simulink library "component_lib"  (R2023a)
settings: Solver=VariableStepAuto  StartTime=0.0  StopTime=10.0  RelTol=1e-3
undefined symbols (not defined in the file or in its folder): component_lib, ECCV_r, KoblenzTrier, mm, par, param_TD04, R1234yf_ph, SigIdentifier, Systems, TH0023_WP120, Thermal, V_nom
libraries: base_lib x166, $bdroot x164, simulink x2, slpidlib x1
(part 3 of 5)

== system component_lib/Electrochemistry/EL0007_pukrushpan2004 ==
  I [A] : Inport
  p_an [Pa x 4] : Inport  Port=2
  p_ca [Pa x 4] : Inport  Port=3
  T_an [K] : Inport  Port=4
  T_ca [K] : Inport  Port=5
  T_fc [K] : Inport  Port=6
  Demux : Demux
  Demux1 : Demux
  F0003_diffusiveFlow.m : base_lib/F0003_pukrushpan2004/F0003_diffusiveFlow.m  SystemSampleTime=-1  VariantActivationTime=update diagram  Latency=0  AutoFrameSizeCalculation=off
  F0003_dragFlow.m : base_lib/F0003_pukrushpan2004/F0003_dragFlow.m  SystemSampleTime=-1  VariantActivationTime=update diagram  Latency=0  AutoFrameSizeCalculation=off
  F0003_outputVoltage.m : base_lib/F0003_pukrushpan2004/F0003_outputVoltage.m  SystemSampleTime=-1  VariantActivationTime=update diagram  Latency=0  AutoFrameSizeCalculation=off
  F0003_reactionFlow.m : base_lib/F0003_pukrushpan2004/F0003_reactionFlow.m  SystemSampleTime=-1  VariantActivationTime=update diagram  Latency=0  AutoFrameSizeCalculation=off
  F0003_vaporActivity.m : base_lib/F0003_pukrushpan2004/F0003_vaporActivity.m  SystemSampleTime=-1  VariantActivationTime=update diagram  Latency=0  AutoFrameSizeCalculation=off
  F0003_vaporActivity.m1 : base_lib/F0003_pukrushpan2004/F0003_vaporActivity.m  SystemSampleTime=-1  VariantActivationTime=update diagram  Latency=0  AutoFrameSizeCalculation=off
  F0003_waterContent.m : base_lib/F0003_pukrushpan2004/F0003_waterContent.m  SystemSampleTime=-1  VariantActivationTime=update diagram  Latency=0  AutoFrameSizeCalculation=off
  F0003_waterContent.m1 : base_lib/F0003_pukrushpan2004/F0003_waterContent.m  SystemSampleTime=-1  VariantActivationTime=update diagram  Latency=0  AutoFrameSizeCalculation=off
  F0010_vaporSaturationPressure.m : base_lib/F0010_gasFlow/F0010_vaporSaturationPressure.m  SystemSampleTime=-1  VariantActivationTime=update diagram  Latency=0  AutoFrameSizeCalculation=off
  F0010_vaporSaturationPressure.m1 : base_lib/F0010_gasFlow/F0010_vaporSaturationPressure.m  SystemSampleTime=-1  VariantActivationTime=update diagram  Latency=0  AutoFrameSizeCalculation=off
  F0010_vaporSaturationPressure.m2 : base_lib/F0010_gasFlow/F0010_vaporSaturationPressure.m  SystemSampleTime=-1  VariantActivationTime=update diagram  Latency=0  AutoFrameSizeCalculation=off
  Gain : Gain  Gain=1/2
  Mux : Mux
  Saturation : Saturate  UpperLimit=inf  LowerLimit=0.01
  Saturation1 : Saturate  UpperLimit=inf  LowerLimit=100
  Saturation2 : Saturate  UpperLimit=inf  LowerLimit=100
  Sum : Sum  Inputs=+|+
  Sum1 : Sum  Inputs=|+-
  Sum2 : Sum  Inputs=|++
  Sum4 : Sum  Inputs=|++
  V [V] : Outport
  W_an [kg/s] : Outport  Port=2
  W_ca [kg/s] : Outport  Port=3
  lam [-] : Outport  Port=4
  Q_gen [J/s] : Outport  Port=5
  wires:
  I [A]/1 -> [I], F0003_reactionFlow.m/1, F0003_outputVoltage.m/1
  F0003_outputVoltage.m/1 -> Saturation/1
  F0003_outputVoltage.m/2 -> Q_gen [J/s]/1
  T_fc [K]/1 -> F0003_diffusiveFlow.m/4, F0010_vaporSaturationPressure.m2/1, F0003_outputVoltage.m/6
  F0010_vaporSaturationPressure.m2/1 -> F0003_outputVoltage.m/4
  F0010_vaporSaturationPressure.m1/1 -> F0003_vaporActivity.m/2
  F0010_vaporSaturationPressure.m/1 -> F0003_vaporActivity.m1/2
  T_an [K]/1 -> F0010_vaporSaturationPressure.m1/1
  T_ca [K]/1 -> F0010_vaporSaturationPressure.m/1
  Demux/3 -> F0003_vaporActivity.m/1
  Demux1/3 -> F0003_vaporActivity.m1/1
  p_an [Pa x 4]/1 -> Demux/1, Saturation1/1
  p_ca [Pa x 4]/1 -> Demux1/1, Saturation2/1
  F0003_vaporActivity.m/1 -> F0003_waterContent.m/1
  F0003_vaporActivity.m1/1 -> F0003_waterContent.m1/1
  F0003_waterContent.m/1 -> Sum/1, F0003_diffusiveFlow.m/1
  F0003_waterContent.m1/1 -> F0003_diffusiveFlow.m/3, Sum/2
  F0003_reactionFlow.m/1 -> Sum1/1
  Sum1/1 -> W_an [kg/s]/1
  F0003_reactionFlow.m/2 -> Sum2/1
  Sum2/1 -> W_ca [kg/s]/1
  [I] -> F0003_dragFlow.m/1
  F0003_diffusiveFlow.m/1 -> Sum4/1
  F0003_dragFlow.m/1 -> Sum4/2
  Mux/1 -> Sum1/2, Sum2/2
  Sum/1 -> Gain/1
  Sum4/1 -> Mux/3
  Saturation/1 -> V [V]/1
  Saturation1/1 -> F0003_outputVoltage.m/2
  Saturation2/1 -> F0003_outputVoltage.m/3
  Gain/1 -> lam [-]/1, F0003_outputVoltage.m/5, F0003_dragFlow.m/2, F0003_diffusiveFlow.m/2

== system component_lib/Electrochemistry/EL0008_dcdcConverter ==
  I_in [A] : Inport
  V_in [V] : Inport  Port=2
  V_bus [V] : Inport  Port=3
  F0020_dcdcConverter.m : base_lib/F0020_dcdcConverter/F0020_dcdcConverter.m  SystemSampleTime=-1  VariantActivationTime=update diagram  Latency=0  AutoFrameSizeCalculation=off
  Terminator : Terminator
  Terminator1 : Terminator
  I_bus [A] : Outport
  Q_gen [J/s] : Outport  Port=2
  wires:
  V_bus [V]/1 -> F0020_dcdcConverter.m/1
  V_in [V]/1 -> F0020_dcdcConverter.m/2
  I_in [A]/1 -> F0020_dcdcConverter.m/3
  F0020_dcdcConverter.m/2 -> I_bus [A]/1
  F0020_dcdcConverter.m/1 -> Terminator/1
  F0020_dcdcConverter.m/4 -> Q_gen [J/s]/1
  F0020_dcdcConverter.m/3 -> Terminator1/1

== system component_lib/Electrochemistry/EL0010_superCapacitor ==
  dI [A] : Inport
  Gain : Gain  Gain=1/C
  Integrator Limited : Integrator  InitialCondition=V_bus0  LimitOutput=on  LowerSaturationLimit=0
  V_bus [V] : Outport
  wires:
  Integrator Limited/1 -> V_bus [V]/1
  dI [A]/1 -> Gain/1
  Gain/1 -> Integrator Limited/1

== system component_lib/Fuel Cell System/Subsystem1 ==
  note: Rolling Fuel Consumption Calculation [kg/100km]
  In1 : Inport
  Add1 : Sum
  Constant6 : Constant
  Constant7 : Constant  Value=100e3
  Demux : Demux
  Divide : Product  Inputs=**/
  Gain1 : Gain  Gain=-1
  Integrator : Integrator
  SC0002_signalRead11 : $bdroot/Data & Control/SC0002_signalRead  SigName=fuelConsumption
  SC0002_signalRead5 : $bdroot/Data & Control/SC0002_signalRead  SigName=hydrogenFlow
  SC0003_signalWrite1 : $bdroot/Data & Control/SC0003_signalWrite  SigName=distance
  Terminator : Terminator
  Terminator1 : Terminator
  Terminator2 : Terminator
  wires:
  Integrator/1 -> Divide/1
  Constant7/1 -> Divide/2
  SC0003_signalWrite1/1 -> Add1/1
  Demux/1 -> Gain1/1
  Add1/1 -> Divide/3
  Constant6/1 -> Add1/2
  Divide/1 -> SC0002_signalRead11/1
  Gain1/1 -> SC0002_signalRead5/1, Integrator/1
  In1/1 -> Demux/1
  Demux/3 -> Terminator1/1
  Demux/4 -> Terminator2/1
  Demux/2 -> Terminator/1

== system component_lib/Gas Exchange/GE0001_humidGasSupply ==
  Constant : Constant  Value=par.p_tot
  Constant1 : Constant  Value=par.RH
  Constant2 : Constant  Value=par.T
  Constant3 : Constant  Value=par.x_H2
  Constant4 : Constant  Value=par.x_O2
  F0010_pressureSupply.m : base_lib/F0010_gasFlow/F0010_pressureSupply.m  SystemSampleTime=-1  VariantActivationTime=update diagram  Latency=0  AutoFrameSizeCalculation=off
  F0010_vaporSaturationPressure.m : base_lib/F0010_gasFlow/F0010_vaporSaturationPressure.m  SystemSampleTime=-1  VariantActivationTime=update diagram  Latency=0  AutoFrameSizeCalculation=off
  p (p x 4) : Outport
  T [K] : Outport  Port=2
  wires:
  Constant2/1 -> T [K]/1, F0010_vaporSaturationPressure.m/1
  Constant/1 -> F0010_pressureSupply.m/1
  F0010_vaporSaturationPressure.m/1 -> F0010_pressureSupply.m/5
  Constant1/1 -> F0010_pressureSupply.m/4
  Constant3/1 -> F0010_pressureSupply.m/2
  Constant4/1 -> F0010_pressureSupply.m/3
  F0010_pressureSupply.m/1 -> p (p x 4)/1

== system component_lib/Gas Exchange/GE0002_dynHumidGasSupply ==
  T [K] : Inport
  p_ref [Pa] : Inport  Port=2
  RH [-] : Inport  Port=3
  Constant : Constant  Value=x_H2_dry
  Constant1 : Constant  Value=x_O2_dry
  F0010_pressureSupply.m : base_lib/F0010_gasFlow/F0010_pressureSupply.m  SystemSampleTime=-1  VariantActivationTime=update diagram  Latency=0  AutoFrameSizeCalculation=off
  F0010_vaporSaturationPressure.m : base_lib/F0010_gasFlow/F0010_vaporSaturationPressure.m  SystemSampleTime=-1  VariantActivationTime=update diagram  Latency=0  AutoFrameSizeCalculation=off
  p (p x 4) : Outport
  T_out [K] : Outport  Port=2
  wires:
  p_ref [Pa]/1 -> F0010_pressureSupply.m/1
  T [K]/1 -> F0010_vaporSaturationPressure.m/1, T_out [K]/1
  F0010_vaporSaturationPressure.m/1 -> F0010_pressureSupply.m/5
  RH [-]/1 -> F0010_pressureSupply.m/4
  F0010_pressureSupply.m/1 -> p (p x 4)/1
  Constant/1 -> F0010_pressureSupply.m/2
  Constant1/1 -> F0010_pressureSupply.m/3

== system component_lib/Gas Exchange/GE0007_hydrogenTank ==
  W_H2 [kg/s] : Inport
  Actuator dynamics : TransferFcn  Denominator=[0.1 1]
  Constant : Constant  Value=0
  Constant2 : Constant  Value=par.V
  Constant3 : Constant  Value=par.T_tank
  Constant4 : Constant  Value=0
  Constant5 : Constant  Value=par.m0
  Constant6 : Constant  Value=par.m0
  Constant7 : Constant  Value=par.M_j(1)
  Constant8 : Constant  Value=par.init_SOC
  Constant9 : Constant  Value=0
  Divide{,1..2,4} (4 alike) : Product  Inputs=*/
  F0005_enthalpy.m : base_lib/F0005_h2Thermodynamics/F0005_enthalpy.m  SystemSampleTime=-1  VariantActivationTime=update diagram  Latency=0  AutoFrameSizeCalculation=off
  F0005_pressure.m : base_lib/F0005_h2Thermodynamics/F0005_pressure.m  SystemSampleTime=-1  VariantActivationTime=update diagram  Latency=0  AutoFrameSizeCalculation=off
  Gain : Gain  Gain=-1
  Hydrogen ideal gas molar specific heat : Constant  Value=par.cp_j(1) .* par.M_j(1);
  Integrator Limited : Integrator  InitialConditionSource=external  LimitOutput=on  LowerSaturationLimit=0
  Mux : Mux
  Product : Product
  Standard state molar enthalpy : Constant  Value=par.h0
  Sum : Sum  Inputs=|+-
  Sum1 : Sum  Inputs=|++
  standard state temperature : Constant  Value=par.T0
  W [kg/s] : Outport
  T [K] : Outport  Port=2
  SOC [-] : Outport  Port=3
  p _tank [Pa] : Outport  Port=4
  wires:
  Integrator Limited/1 -> Divide1/1, Divide2/1
  Constant2/1 -> Divide1/2
  Constant3/1 -> F0005_pressure.m/1, F0005_enthalpy.m/1
  F0005_pressure.m/1 -> p _tank [Pa]/1
  Divide2/1 -> SOC [-]/1
  Hydrogen ideal gas molar specific heat/1 -> Divide/2
  Divide1/1 -> Divide4/1
  Constant7/1 -> Divide4/2
  Divide4/1 -> F0005_enthalpy.m/2, F0005_pressure.m/2
  F0005_enthalpy.m/1 -> Sum/1
  Standard state molar enthalpy/1 -> Sum/2
  Sum/1 -> Divide/1
  Divide/1 -> Sum1/1
  standard state temperature/1 -> Sum1/2
  Sum1/1 -> T [K]/1
  Constant5/1 -> Divide2/2
  Constant6/1 -> Product/1
  Product/1 -> Integrator Limited/2
  Constant8/1 -> Product/2
  Constant9/1 -> Mux/4
  Constant/1 -> Mux/2
  Constant4/1 -> Mux/3
  Actuator dynamics/1 -> Gain/1, Mux/1
  Mux/1 -> W [kg/s]/1
  Gain/1 -> Integrator Limited/1
  W_H2 [kg/s]/1 -> Actuator dynamics/1

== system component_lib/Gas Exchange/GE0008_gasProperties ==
  p (p x 4) : Inport
  T [K] : Inport  Port=2
  Demux : Demux
  Divide : Product  Inputs=*/
  F0010_vaporSaturationPressure.m : base_lib/F0010_gasFlow/F0010_vaporSaturationPressure.m  SystemSampleTime=-1  VariantActivationTime=update diagram  Latency=0  AutoFrameSizeCalculation=off
  Mux : Mux
  Sum : Sum  Inputs=|+|
  p [Pa] : Outport
  RH [-] : Outport  Port=2
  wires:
  Sum/1 -> p [Pa]/1
  p (p x 4)/1 -> Demux/1
  Demux/1 -> Mux/1
  Demux/2 -> Mux/2
  Demux/3 -> Divide/1, Mux/3
  Demux/4 -> Mux/4
  Mux/1 -> Sum/1
  Divide/1 -> RH [-]/1
  F0010_vaporSaturationPressure.m/1 -> Divide/2
  T [K]/1 -> F0010_vaporSaturationPressure.m/1

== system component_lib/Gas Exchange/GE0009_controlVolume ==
  note: Pressure
  note: Mass flow contribution to pressure dynamics
  dW [kg/s x 4] : Inport
  T [K] : Inport  Port=2
  Constant : Constant  Value=par.p0
  Constant1 : Constant  Value=par.RH0
  Constant3 : Constant  Value=par.V
  Constant5 : Constant  Value=par.x0_H2
  Constant6 : Constant  Value=par.x0_O2
  Divide1 : Product  Inputs=***/
  F0010_pressureSupply.m : base_lib/F0010_gasFlow/F0010_pressureSupply.m  SystemSampleTime=-1  VariantActivationTime=update diagram  Latency=0  AutoFrameSizeCalculation=off
  F0010_vaporSaturationPressure.m : base_lib/F0010_gasFlow/F0010_vaporSaturationPressure.m  SystemSampleTime=-1  VariantActivationTime=update diagram  Latency=0  AutoFrameSizeCalculation=off
  Gas constants : Constant  Value=par.R_j
  Integrator Limited1 : Integrator  InitialConditionSource=external  LimitOutput=on  LowerSaturationLimit=0
  p [Pa x 4] : Outport
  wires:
  Integrator Limited1/1 -> p [Pa x 4]/1
  Constant/1 -> F0010_pressureSupply.m/1
  F0010_pressureSupply.m/1 -> Integrator Limited1/2
  dW [kg/s x 4]/1 -> Divide1/1
  Divide1/1 -> Integrator Limited1/1
  Constant3/1 -> Divide1/4
  Gas constants/1 -> Divide1/2
  F0010_vaporSaturationPressure.m/1 -> F0010_pressureSupply.m/5
  Constant1/1 -> F0010_pressureSupply.m/4
  Constant5/1 -> F0010_pressureSupply.m/2
  Constant6/1 -> F0010_pressureSupply.m/3
  T [K]/1 -> F0010_vaporSaturationPressure.m/1, Divide1/3

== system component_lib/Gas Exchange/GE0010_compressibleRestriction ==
  p_us [Pa x 4] : Inport
  T_us [K] : Inport  Port=2
  p_ds [Pa x 4] : Inport  Port=3
  Area : Constant  Value=pi*(D_t/2)^2
  F0010_compressibleRestriction.m : base_lib/F0010_gasFlow/F0010_compressibleRestriction.m  SystemSampleTime=-1  VariantActivationTime=update diagram  Latency=0  AutoFrameSizeCalculation=off
  F0010_mixtureProperties.m : base_lib/F0010_gasFlow/F0010_mixtureProperties.m  SystemSampleTime=-1  VariantActivationTime=update diagram  Latency=0  AutoFrameSizeCalculation=off
  F0010_multicomponentFlow.m : base_lib/F0010_gasFlow/F0010_multicomponentFlow.m  SystemSampleTime=-1  VariantActivationTime=update diagram  Latency=0  AutoFrameSizeCalculation=off
  Sum : Sum  Inputs=+
  Sum1 : Sum  Inputs=+
  Terminator : Terminator
  Terminator1 : Terminator
  W [kg/s x 4] : Outport
  T_ds [K] : Outport  Port=2
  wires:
  T_us [K]/1 -> F0010_compressibleRestriction.m/3, T_ds [K]/1
  p_us [Pa x 4]/1 -> Sum/1, F0010_mixtureProperties.m/1, F0010_multicomponentFlow.m/1
  p_ds [Pa x 4]/1 -> Sum1/1
  Sum/1 -> F0010_compressibleRestriction.m/1
  Sum1/1 -> F0010_compressibleRestriction.m/2
  F0010_compressibleRestriction.m/1 -> F0010_multicomponentFlow.m/2
  F0010_multicomponentFlow.m/1 -> W [kg/s x 4]/1
  F0010_mixtureProperties.m/2 -> F0010_compressibleRestriction.m/4
  F0010_mixtureProperties.m/4 -> F0010_compressibleRestriction.m/5
  F0010_mixtureProperties.m/1 -> Terminator/1
  F0010_mixtureProperties.m/3 -> Terminator1/1
  Area/1 -> F0010_compressibleRestriction.m/6

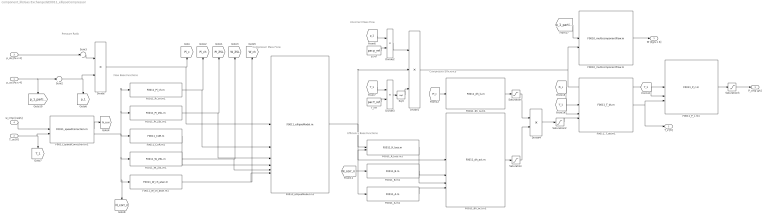
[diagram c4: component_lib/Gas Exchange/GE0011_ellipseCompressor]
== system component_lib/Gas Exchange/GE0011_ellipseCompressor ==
  note: Compressor Mass FLow
  note: Compressor Efficiency
  note: Efficiency Base Functions
  note: Pressure Ratio
  note: Flow Base Functions
  note: Uncorrect Mass Flow
  p_us [Pa x 4] : Inport
  T_us [K] : Inport  Port=2
  p_ds [Pa x 4] : Inport  Port=3
  w_cmp [rad/s] : Inport  Port=4
  Divide{,2..4} (4 alike) : Product  Inputs=*/
  Divide1 : Product  Inputs=**/
  F0010_multicomponentFlow.m : base_lib/F0010_gasFlow/F0010_multicomponentFlow.m  SystemSampleTime=-1  VariantActivationTime=update diagram  Latency=0  AutoFrameSizeCalculation=off
  F0011_A.m1 : base_lib/F0011_ellipseCompressor/F0011_A.m  SystemSampleTime=-1  VariantActivationTime=update diagram  Latency=0  AutoFrameSizeCalculation=off
  F0011_B.m1 : base_lib/F0011_ellipseCompressor/F0011_B.m  SystemSampleTime=-1  VariantActivationTime=update diagram  Latency=0  AutoFrameSizeCalculation=off
  F0011_CUR.m1 : base_lib/F0011_ellipseCompressor/F0011_CUR.m  SystemSampleTime=-1  VariantActivationTime=update diagram  Latency=0  AutoFrameSizeCalculation=off
  F0011_K_loss.m1 : base_lib/F0011_ellipseCompressor/F0011_K_loss.m  SystemSampleTime=-1  VariantActivationTime=update diagram  Latency=0  AutoFrameSizeCalculation=off
  F0011_PI_ZSL.m1 : base_lib/F0011_ellipseCompressor/F0011_PI_ZSL.m  SystemSampleTime=-1  VariantActivationTime=update diagram  Latency=0  AutoFrameSizeCalculation=off
  F0011_P_c.m1 : base_lib/F0011_ellipseCompressor/F0011_P_c.m  SystemSampleTime=-1  VariantActivationTime=update diagram  Latency=0  AutoFrameSizeCalculation=off
  F0011_Pi_ch.m1 : base_lib/F0011_ellipseCompressor/F0011_Pi_ch.m  SystemSampleTime=-1  VariantActivationTime=update diagram  Latency=0  AutoFrameSizeCalculation=off
  F0011_T_ds.m1 : base_lib/F0011_ellipseCompressor/F0011_T_ds.m  SystemSampleTime=-1  VariantActivationTime=update diagram  Latency=0  AutoFrameSizeCalculation=off
  F0011_W_ZSL.m1 : base_lib/F0011_ellipseCompressor/F0011_W_ZSL.m  SystemSampleTime=-1  VariantActivationTime=update diagram  Latency=0  AutoFrameSizeCalculation=off
  F0011_W_ch_atan.m1 : base_lib/F0011_ellipseCompressor/F0011_W_ch_atan.m  SystemSampleTime=-1  VariantActivationTime=update diagram  Latency=0  AutoFrameSizeCalculation=off
  F0011_dh_act.m1 : base_lib/F0011_ellipseCompressor/F0011_dh_act.m  SystemSampleTime=-1  VariantActivationTime=update diagram  Latency=0  AutoFrameSizeCalculation=off
  F0011_dh_is.m1 : base_lib/F0011_ellipseCompressor/F0011_dh_is.m  SystemSampleTime=-1  VariantActivationTime=update diagram  Latency=0  AutoFrameSizeCalculation=off
  F0011_ellipseModel.m1 : base_lib/F0011_ellipseCompressor/F0011_ellipseModel.m  SystemSampleTime=-1  VariantActivationTime=update diagram  Latency=0  AutoFrameSizeCalculation=off
  F0011_speedCorrection.m1 : base_lib/F0011_ellipseCompressor/F0011_speedCorrection.m  SystemSampleTime=-1  VariantActivationTime=update diagram  Latency=0  AutoFrameSizeCalculation=off
  Saturation : Saturate  UpperLimit=inf  LowerLimit=1e-4
  Saturation1 : Saturate  UpperLimit=inf  LowerLimit=1e-4
  Saturation2 : Saturate  UpperLimit=1  LowerLimit=1e-3
  Saturation3 : Saturate  UpperLimit=inf  LowerLimit=0
  Sqrt : Sqrt
  Sum2 : Sum  Inputs=|+|
  Sum3 : Sum  Inputs=|+|
  T_ref : Constant  Value=par.T_ref
  p_ref : Constant  Value=par.p_ref
  W [kg/s x 4] : Outport
  T_2 [K] : Outport  Port=2
  P_cmp [J/s] : Outport  Port=3
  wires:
  Sum3/1 -> Divide/1
  T_us [K]/1 -> F0011_speedCorrection.m1/2, [T_1]
  F0011_CUR.m1/1 -> F0011_ellipseModel.m1/4
  F0011_PI_ZSL.m1/1 -> F0011_ellipseModel.m1/3, [PI_ZSL]
  F0011_W_ZSL.m1/1 -> F0011_ellipseModel.m1/5, [W_ZSL]
  F0011_W_ch_atan.m1/1 -> F0011_ellipseModel.m1/6, [W_ch]
  F0011_speedCorrection.m1/2 -> F0011_CUR.m1/1, F0011_W_ZSL.m1/1, F0011_W_ch_atan.m1/1, [N_corr_n], F0011_PI_ZSL.m1/1, F0011_Pi_ch.m1/1
  Divide/1 -> F0011_ellipseModel.m1/1, [Pi_c]
  F0011_speedCorrection.m1/1 -> [N_corr]
  Divide1/1 -> F0011_P_c.m1/1, F0010_multicomponentFlow.m/2
  p_ref/1 -> Divide2/2
  Divide2/1 -> Divide1/1
  [p_1] -> Divide2/1
  [T_1] -> Divide3/1
  T_ref/1 -> Divide3/2
  Divide3/1 -> Sqrt/1
  Sqrt/1 -> Divide1/3
  F0011_Pi_ch.m1/1 -> F0011_ellipseModel.m1/2, [Pi_ch]
  F0011_K_loss.m1/1 -> F0011_dh_act.m1/2
  F0011_B.m1/1 -> F0011_dh_act.m1/3
  F0011_A.m1/1 -> F0011_dh_act.m1/4
  [N_corr_n] -> F0011_A.m1/1, F0011_B.m1/1, F0011_K_loss.m1/2
  [Pi_c] -> F0011_dh_is.m1/1
  F0011_dh_act.m1/1 -> Saturation/1
  F0011_dh_is.m1/1 -> Saturation1/1
  Saturation1/1 -> Divide4/1
  Saturation/1 -> Divide4/2
  Divide4/1 -> Saturation2/1
  Saturation2/1 -> F0011_T_ds.m1/3
  F0011_T_ds.m1/1 -> F0011_P_c.m1/3, T_2 [K]/1
  [T_1] -> F0011_P_c.m1/2
  [T_1] -> F0011_T_ds.m1/2
  [Pi_c] -> F0011_T_ds.m1/1
  w_cmp [rad/s]/1 -> F0011_speedCorrection.m1/1
  p_us [Pa x 4]/1 -> Sum2/1, [p_1_partial]
  Sum2/1 -> Divide/2, [p_1]
  [p_1_partial] -> F0010_multicomponentFlow.m/1
  F0010_multicomponentFlow.m/1 -> W [kg/s x 4]/1
  F0011_ellipseModel.m1/1 -> F0011_dh_act.m1/1, F0011_K_loss.m1/1, Divide1/2
  p_ds [Pa x 4]/1 -> Sum3/1
  F0011_P_c.m1/1 -> Saturation3/1
  Saturation3/1 -> P_cmp [J/s]/1

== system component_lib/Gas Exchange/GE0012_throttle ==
  p_us [Pa x 4] : Inport
  T_us [K] : Inport  Port=2
  p_ds [Pa x 4] : Inport  Port=3
  alpha [-] : Inport  Port=4
  F0010_compressibleRestriction.m : base_lib/F0010_gasFlow/F0010_compressibleRestriction.m  SystemSampleTime=-1  VariantActivationTime=update diagram  Latency=0  AutoFrameSizeCalculation=off
  F0010_mixtureProperties.m : base_lib/F0010_gasFlow/F0010_mixtureProperties.m  SystemSampleTime=-1  VariantActivationTime=update diagram  Latency=0  AutoFrameSizeCalculation=off
  F0010_multicomponentFlow.m : base_lib/F0010_gasFlow/F0010_multicomponentFlow.m  SystemSampleTime=-1  VariantActivationTime=update diagram  Latency=0  AutoFrameSizeCalculation=off
  F0010_throttleArea.m : base_lib/F0010_gasFlow/F0010_throttleArea.m  SystemSampleTime=-1  VariantActivationTime=update diagram  Latency=0  AutoFrameSizeCalculation=off
  Sum : Sum  Inputs=+
  Sum1 : Sum  Inputs=+
  Terminator : Terminator
  Terminator1 : Terminator
  W [kg/s x 4] : Outport
  T_out [K] : Outport  Port=2
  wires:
  T_us [K]/1 -> F0010_compressibleRestriction.m/3, T_out [K]/1
  p_us [Pa x 4]/1 -> Sum/1, F0010_mixtureProperties.m/1, F0010_multicomponentFlow.m/1
  p_ds [Pa x 4]/1 -> Sum1/1
  Sum/1 -> F0010_compressibleRestriction.m/1
  Sum1/1 -> F0010_compressibleRestriction.m/2
  F0010_compressibleRestriction.m/1 -> F0010_multicomponentFlow.m/2
  F0010_multicomponentFlow.m/1 -> W [kg/s x 4]/1
  F0010_mixtureProperties.m/2 -> F0010_compressibleRestriction.m/4
  F0010_mixtureProperties.m/4 -> F0010_compressibleRestriction.m/5
  F0010_mixtureProperties.m/1 -> Terminator/1
  F0010_mixtureProperties.m/3 -> Terminator1/1
  F0010_throttleArea.m/1 -> F0010_compressibleRestriction.m/6
  alpha [-]/1 -> F0010_throttleArea.m/1

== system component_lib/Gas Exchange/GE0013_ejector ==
  p_p [Pa x 4] : Inport
  T_p [K] : Inport  Port=2
  p_s [Pa x 4] : Inport  Port=3
  T_s [K] : Inport  Port=4
  p_b [Pa x 4] : Inport  Port=5
  Divide : Product  Inputs=*/
  F0010_ejectorModel.m : base_lib/F0010_gasFlow/F0010_ejectorModel.m  SystemSampleTime=-1  VariantActivationTime=update diagram  Latency=0  AutoFrameSizeCalculation=off
  F0010_multicomponentFlow.m : base_lib/F0010_gasFlow/F0010_multicomponentFlow.m  SystemSampleTime=-1  VariantActivationTime=update diagram  Latency=0  AutoFrameSizeCalculation=off
  F0010_multicomponentFlow.m1 : base_lib/F0010_gasFlow/F0010_multicomponentFlow.m  SystemSampleTime=-1  VariantActivationTime=update diagram  Latency=0  AutoFrameSizeCalculation=off
  F0010_vaporSaturationPressure.m : base_lib/F0010_gasFlow/F0010_vaporSaturationPressure.m  SystemSampleTime=-1  VariantActivationTime=update diagram  Latency=0  AutoFrameSizeCalculation=off
  Selector : Selector  InputPortWidth=4  IndexOptions=Index vector (dialog)  Indices=3  OutputSizes=1
  Sum : Sum  Inputs=+
  Sum1 : Sum  Inputs=+
  Sum2 : Sum  Inputs=+
  W_p [kg/s] : Outport
  W_s [kg/s] : Outport  Port=2
  phi [-] : Outport  Port=3
  w [-] : Outport  Port=4
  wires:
  p_p [Pa x 4]/1 -> Sum/1, [P_p]
  Sum/1 -> F0010_ejectorModel.m/1
  p_s [Pa x 4]/1 -> Sum1/1, [P_s]
  Sum1/1 -> F0010_ejectorModel.m/2
  Sum2/1 -> F0010_ejectorModel.m/3
  p_b [Pa x 4]/1 -> Sum2/1
  F0010_ejectorModel.m/1 -> F0010_multicomponentFlow.m/2
  F0010_multicomponentFlow.m/1 -> W_p [kg/s]/1
  F0010_ejectorModel.m/2 -> F0010_multicomponentFlow.m1/2
  F0010_multicomponentFlow.m1/1 -> W_s [kg/s]/1
  [P_p] -> F0010_multicomponentFlow.m/1
  [P_s] -> F0010_multicomponentFlow.m1/1
  F0010_ejectorModel.m/3 -> phi [-]/1
  T_p [K]/1 -> F0010_ejectorModel.m/4, [T_p]
  T_s [K]/1 -> F0010_vaporSaturationPressure.m/1
  [P_s] -> Selector/1
  Divide/1 -> F0010_ejectorModel.m/6
  Selector/1 -> Divide/1
  F0010_vaporSaturationPressure.m/1 -> F0010_ejectorModel.m/5, Divide/2
  F0010_ejectorModel.m/4 -> w [-]/1

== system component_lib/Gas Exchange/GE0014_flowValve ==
  p_us [Pa x 4] : Inport
  T_us [K] : Inport  Port=2
  p_ds [Pa x 4] : Inport  Port=3
  open [-] : Inport  Port=4
  Area : Constant  Value=pi*(D_t/2)^2
  F0010_compressibleRestriction.m : base_lib/F0010_gasFlow/F0010_compressibleRestriction.m  SystemSampleTime=-1  VariantActivationTime=update diagram  Latency=0  AutoFrameSizeCalculation=off
  F0010_mixtureProperties.m : base_lib/F0010_gasFlow/F0010_mixtureProperties.m  SystemSampleTime=-1  VariantActivationTime=update diagram  Latency=0  AutoFrameSizeCalculation=off
  F0010_multicomponentFlow.m : base_lib/F0010_gasFlow/F0010_multicomponentFlow.m  SystemSampleTime=-1  VariantActivationTime=update diagram  Latency=0  AutoFrameSizeCalculation=off
  Product : Product
  Sum : Sum  Inputs=+
  Sum1 : Sum  Inputs=+
  Terminator : Terminator
  Terminator1 : Terminator
  W [kg/s x 4] : Outport
  T_ds [K] : Outport  Port=2
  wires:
  T_us [K]/1 -> F0010_compressibleRestriction.m/3, T_ds [K]/1
  p_us [Pa x 4]/1 -> Sum/1, F0010_mixtureProperties.m/1, F0010_multicomponentFlow.m/1
  p_ds [Pa x 4]/1 -> Sum1/1
  Sum/1 -> F0010_compressibleRestriction.m/1
  Sum1/1 -> F0010_compressibleRestriction.m/2
  F0010_compressibleRestriction.m/1 -> F0010_multicomponentFlow.m/2
  F0010_multicomponentFlow.m/1 -> W [kg/s x 4]/1
  F0010_mixtureProperties.m/2 -> F0010_compressibleRestriction.m/4
  F0010_mixtureProperties.m/4 -> F0010_compressibleRestriction.m/5
  F0010_mixtureProperties.m/1 -> Terminator/1
  F0010_mixtureProperties.m/3 -> Terminator1/1
  Area/1 -> Product/1
  Product/1 -> F0010_compressibleRestriction.m/6
  open [-]/1 -> Product/2

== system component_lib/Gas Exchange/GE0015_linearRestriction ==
  p_us [Pa x 4] : Inport
  p_ds [Pa x 4] : Inport  Port=2
  F0010_linearRestriction.m : base_lib/F0010_gasFlow/F0010_linearRestriction.m  SystemSampleTime=-1  VariantActivationTime=update diagram  Latency=0  AutoFrameSizeCalculation=off
  F0010_multicomponentFlow.m : base_lib/F0010_gasFlow/F0010_multicomponentFlow.m  SystemSampleTime=-1  VariantActivationTime=update diagram  Latency=0  AutoFrameSizeCalculation=off
  Sum : Sum  Inputs=+
  Sum1 : Sum  Inputs=+
  W [kg/s x 4] : Outport
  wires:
  F0010_multicomponentFlow.m/1 -> W [kg/s x 4]/1
  p_us [Pa x 4]/1 -> F0010_multicomponentFlow.m/1, Sum/1
  p_ds [Pa x 4]/1 -> Sum1/1
  Sum/1 -> F0010_linearRestriction.m/1
  Sum1/1 -> F0010_linearRestriction.m/2
  F0010_linearRestriction.m/1 -> F0010_multicomponentFlow.m/2

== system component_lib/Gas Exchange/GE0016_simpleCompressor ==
  W [kg/s] : Inport
  p2 [Pa] : Inport  Port=2
  T1 [K] : Inport  Port=3
  p1 [Pa] : Inport  Port=4
  Constant : Constant  Value=eta
  F0007_compressorPower.m : base_lib/F0019_simpleCompressor/F0007_compressorPower.m  SystemSampleTime=-1  VariantActivationTime=update diagram  Latency=0  AutoFrameSizeCalculation=off
  F0007_compressorTemperature.m : base_lib/F0019_simpleCompressor/F0007_compressorTemperature.m  SystemSampleTime=-1  VariantActivationTime=update diagram  Latency=0  AutoFrameSizeCalculation=off
  P_cmp [J/s] : Outport
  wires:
  T1 [K]/1 -> F0007_compressorTemperature.m/3, F0007_compressorPower.m/2
  F0007_compressorTemperature.m/1 -> F0007_compressorPower.m/3
  W [kg/s]/1 -> F0007_compressorPower.m/1
  F0007_compressorPower.m/1 -> P_cmp [J/s]/1
  Constant/1 -> F0007_compressorTemperature.m/4
  p2 [Pa]/1 -> F0007_compressorTemperature.m/2
  p1 [Pa]/1 -> F0007_compressorTemperature.m/1

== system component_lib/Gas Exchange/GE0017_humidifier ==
  p [Pa x 4]) : Inport
  RH_ref [-] : Inport  Port=2
  T [K] : Inport  Port=3
  Demux : Demux
  F0003_vaporActivity.m : base_lib/F0003_pukrushpan2004/F0003_vaporActivity.m  SystemSampleTime=-1  VariantActivationTime=update diagram  Latency=0  AutoFrameSizeCalculation=off
  F0010_vaporSaturationPressure.m : base_lib/F0010_gasFlow/F0010_vaporSaturationPressure.m  SystemSampleTime=-1  VariantActivationTime=update diagram  Latency=0  AutoFrameSizeCalculation=off
  Gain : Gain  Gain=gain
  Mux : Mux
  Sum : Sum  Inputs=|+-
  W [kg/s x 4] : Outport
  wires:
  Sum/1 -> Gain/1
  F0010_vaporSaturationPressure.m/1 -> F0003_vaporActivity.m/2
  Demux/3 -> F0003_vaporActivity.m/1
  Gain/1 -> Mux/3
  p [Pa x 4])/1 -> Demux/1
  T [K]/1 -> F0010_vaporSaturationPressure.m/1
  Mux/1 -> W [kg/s x 4]/1
  F0003_vaporActivity.m/1 -> Sum/2
  RH_ref [-]/1 -> Sum/1

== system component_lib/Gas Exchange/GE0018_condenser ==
  p_in [Pa x 4]) : Inport
  T_cds [K] : Inport  Port=2
  Constant : Constant
  Demux : Demux
  F0003_vaporActivity.m : base_lib/F0003_pukrushpan2004/F0003_vaporActivity.m  SystemSampleTime=-1  VariantActivationTime=update diagram  Latency=0  AutoFrameSizeCalculation=off
  F0010_vaporSaturationPressure.m : base_lib/F0010_gasFlow/F0010_vaporSaturationPressure.m  SystemSampleTime=-1  VariantActivationTime=update diagram  Latency=0  AutoFrameSizeCalculation=off
  Gain : Gain  Gain=gain
  Mux : Mux
  Saturation : Saturate  UpperLimit=inf  LowerLimit=0  ZeroCross=off
  Sum : Sum  Inputs=|+-
  W [kg/s x 4] : Outport
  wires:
  Demux/3 -> F0003_vaporActivity.m/1
  p_in [Pa x 4])/1 -> Demux/1
  F0010_vaporSaturationPressure.m/1 -> F0003_vaporActivity.m/2
  T_cds [K]/1 -> F0010_vaporSaturationPressure.m/1
  Constant/1 -> Sum/2
  Mux/1 -> W [kg/s x 4]/1
  Saturation/1 -> Gain/1
  Sum/1 -> Saturation/1
  Gain/1 -> Mux/3
  F0003_vaporActivity.m/1 -> Sum/1

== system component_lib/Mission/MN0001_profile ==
  v [m/s] : Inport
  Altitute lookup table : Lookup_n-D  NumberOfTableDimensions=1  BreakpointsForDimension1=ECCV_r.distance  Table=ECCV_r.altitude  InternalRulePriority=Speed  RndMeth=Simplest
  Compare To Constant : simulink/Logic and Bit Operations/Compare To Constant  relop=>=  const=ECCV_r.distance(end)  OutDataTypeStr=boolean
  Constant1 : Constant  Value=ECCV_r.slope
  Find current index of distance vector : Lookup_n-D  NumberOfTableDimensions=1  BreakpointsForDimension1=ECCV_r.distance  Table=1:length(ECCV_r.distance)  InterpMethod=Nearest  InternalRulePriority=Speed  RndMeth=Simplest
  Initial position : Constant  Value=x0
  Integrator1 : Integrator  InitialConditionSource=external
  Selector : Selector  InputPortWidth=length(ECCV_r.slope)  IndexOptions=Starting index (port)  Indices=[1 3]  OutputSizes=N_lookahead
  Slope lookup table : Lookup_n-D  NumberOfTableDimensions=1  BreakpointsForDimension1=ECCV_r.distance  Table=ECCV_r.slope  InternalRulePriority=Speed  RndMeth=Simplest
  Stop Simulation : Stop
  slope [rad] : Outport
  altitude [m] : Outport  Port=2
  distance [m] : Outport  Port=3
  slope_lookahead [rad] : Outport  Port=4
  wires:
  Integrator1/1 -> Find current index of distance vector/1, Altitute lookup table/1, Slope lookup table/1, distance [m]/1, Compare To Constant/1
  Slope lookup table/1 -> slope [rad]/1
  Altitute lookup table/1 -> altitude [m]/1
  Compare To Constant/1 -> Stop Simulation/1
  Selector/1 -> slope_lookahead [rad]/1
  Constant1/1 -> Selector/1
  Find current index of distance vector/1 -> Selector/2
  Initial position/1 -> Integrator1/2
  v [m/s]/1 -> Integrator1/1

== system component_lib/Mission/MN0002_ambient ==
  note: 4 % per km decrease
  altitude [m] : Inport
  Constant : Constant  Value=RH_0
  F0018_troposphereModel.m : base_lib/F0018_ambientProperties/F0018_troposphereModel.m  SystemSampleTime=-1  VariantActivationTime=update diagram  Latency=0  AutoFrameSizeCalculation=off
  Gain : Gain  Gain=0.04e-3
  Product : Product
  Sum : Sum  Inputs=|+-
  T [K] : Outport
  p [Pa] : Outport  Port=2
  RH [-] : Outport  Port=3
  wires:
  F0018_troposphereModel.m/2 -> T [K]/1
  F0018_troposphereModel.m/1 -> p [Pa]/1
  altitude [m]/1 -> Gain/1, F0018_troposphereModel.m/1
  Gain/1 -> Product/2
  Constant/1 -> Sum/1, Product/1
  Product/1 -> Sum/2
  Sum/1 -> RH [-]/1

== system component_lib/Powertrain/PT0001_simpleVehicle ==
  note: Tractive force
  Tq_in [Nm] : Inport
  alpha [rad] : Inport  Port=2
  brake [-] : Inport  Port=3
  Abs : Abs
  Abs1 : Abs
  Constant : Constant  Value=par.r_w
  Divide : Product  Inputs=*/
  Divide1 : Product  Inputs=*/
  F0006_airDrag.m : base_lib/F0006_truckBenchmark/F0006_airDrag.m  SystemSampleTime=-1  VariantActivationTime=update diagram  Latency=0  AutoFrameSizeCalculation=off
  F0006_brakeForce.m : base_lib/F0006_truckBenchmark/F0006_brakeForce.m  SystemSampleTime=-1  VariantActivationTime=update diagram  Latency=0  AutoFrameSizeCalculation=off
  F0006_gravitationalForce.m : base_lib/F0006_truckBenchmark/F0006_gravitationalForce.m  SystemSampleTime=-1  VariantActivationTime=update diagram  Latency=0  AutoFrameSizeCalculation=off
  F0006_rollingResistance.m : base_lib/F0006_truckBenchmark/F0006_rollingResistance.m  SystemSampleTime=-1  VariantActivationTime=update diagram  Latency=0  AutoFrameSizeCalculation=off
  Gain : Gain  Gain=1/par.m
  Initial speed : Constant  Value=par.v0
  Integrator2 : Integrator  InitialConditionSource=external
  Sum : Sum  Inputs=+++
  Sum1 : Sum  Inputs=|+-
  Sum2 : Sum  Inputs=++|
  v [m/s] : Outport
  w_w [rad/s] : Outport  Port=2
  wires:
  alpha [rad]/1 -> F0006_gravitationalForce.m/1, F0006_rollingResistance.m/2
  Initial speed/1 -> Integrator2/2
  F0006_airDrag.m/1 -> Sum/1
  F0006_rollingResistance.m/1 -> Sum/2
  Sum1/1 -> Gain/1
  F0006_gravitationalForce.m/1 -> Sum/3
  Gain/1 -> Integrator2/1
  Sum2/1 -> Sum1/2
  Sum/1 -> Sum2/2
  Integrator2/1 -> Divide1/1, Abs1/1, Abs/1, v [m/s]/1
  Abs/1 -> F0006_airDrag.m/1
  Abs1/1 -> F0006_rollingResistance.m/1
  Divide1/1 -> w_w [rad/s]/1
  brake [-]/1 -> F0006_brakeForce.m/1
  F0006_brakeForce.m/1 -> Sum2/1
  Divide/1 -> Sum1/1
  Tq_in [Nm]/1 -> Divide/1
  Constant/1 -> Divide/2, Divide1/2

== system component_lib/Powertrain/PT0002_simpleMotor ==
  Tq_ref [Nm] : Inport
  V [V] : Inport  Port=2
  w_em [rad/s] : Inport  Port=3
  F0009_currentDemand.m : base_lib/F0009_simpleTractionMotor/F0009_currentDemand.m  SystemSampleTime=-1  VariantActivationTime=update diagram  Latency=0  AutoFrameSizeCalculation=off
  Torque dynamics : TransferFcn  Denominator=[T_s 1]
  Tq_em [Nm] : Outport
  I_em [A] : Outport  Port=2
  Q_gen [J/s] : Outport  Port=3
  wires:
  w_em [rad/s]/1 -> F0009_currentDemand.m/3
  V [V]/1 -> F0009_currentDemand.m/2
  Torque dynamics/1 -> Tq_em [Nm]/1, F0009_currentDemand.m/1
  Tq_ref [Nm]/1 -> Torque dynamics/1
  F0009_currentDemand.m/2 -> I_em [A]/1
  F0009_currentDemand.m/1 -> Q_gen [J/s]/1

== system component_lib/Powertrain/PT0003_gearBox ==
  Tq_in [Nm] : Inport
  w_out [rad/s] : Inport  Port=2
  gear  [-] : Inport  Port=3
  clutch  [-] : Inport  Port=4
  1-D Lookup Table : Lookup_n-D  NumberOfTableDimensions=1  BreakpointsForDimension1=par.gears  Table=par.gear_ratios  InterpMethod=Nearest  InternalRulePriority=Speed  RndMeth=Simplest
  F0006_gearBox.m : base_lib/F0006_truckBenchmark/F0006_gearBox.m  SystemSampleTime=-1  VariantActivationTime=update diagram  Latency=0  AutoFrameSizeCalculation=off
  Product : Product
  Tq_out [Nm] : Outport
  w_in [rad/s] : Outport  Port=2
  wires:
  w_out [rad/s]/1 -> F0006_gearBox.m/2
  Tq_in [Nm]/1 -> F0006_gearBox.m/1
  F0006_gearBox.m/2 -> w_in [rad/s]/1
  1-D Lookup Table/1 -> F0006_gearBox.m/3
  gear  [-]/1 -> 1-D Lookup Table/1
  clutch  [-]/1 -> Product/1
  F0006_gearBox.m/1 -> Product/2
  Product/1 -> Tq_out [Nm]/1

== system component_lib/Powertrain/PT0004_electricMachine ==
  I [A] : Inport
  V [V] : Inport  Port=2
  w [rad/s] : Inport  Port=3
  Abs : Abs
  Abs1 : Abs
  Abs2 : Abs
  Constant1 : Constant  Value=V_nom
  Divide : Product  Inputs=**/
  F0009_torque.m : base_lib/F0009_simpleTractionMotor/F0009_torque.m  SystemSampleTime=-1  VariantActivationTime=update diagram  Latency=0  AutoFrameSizeCalculation=off
  Gain : Gain  Gain=-1
  Product : Product
  Product1 : Product
  Sum : Sum  Inputs=|+-
  Torque Limiter : simulink/Discontinuities/Saturation Dynamic  OutMin=[]  OutMax=[]  OutDataTypeStr=Inherit: Same as second input  OutDataType=fixdt(1, 16)  OutScaling=2^-10  DoSatur=off
  "[0, V_nom]" : Saturate  UpperLimit=V_nom  LowerLimit=0
  "[0,476]" : Saturate  UpperLimit=476  LowerLimit=0
  speed-Torque map1 : Lookup_n-D  NumberOfTableDimensions=1  BreakpointsForDimension1=|  Table=|  ExtrapMethod=Clip  UseLastTableValue=on  InternalRulePriority=Speed  RndMeth=Simplest
      | [25.2590673575129
      | 34.9740932642487
      | 43.3937823834197
      | 51.1658031088083
      | 55.6994818652850
      | 64.1191709844560
      | 65.4145077720207
      | 67.3575129533679
      | 68.0051813471503
      | 69.9481865284974
      | 71.2435233160622
      | 73.1865284974093
      | 75.7772020725389
      | 76.4248704663213
      | 78.3678756476684
      | 81.6062176165803
      | 82.9015544041451
      | 86.1398963730570
      | 88.0829015544041
      | 90.0259067357513
      | 94.5595854922280
      | 97.1502590673575
      | 100.388601036269
      | 103.6269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
      | [1991.26637554585
      | 1997.08879184862
      | 1994.17758369723
      | 1994.17758369723
      | 1994.17758369723
      | 1991.26637554585
      | 1944.68704512373
      | 1921.39737991266
      | 1854.43959243086
      | 1816.59388646288
      | 1787.48180494905
      | 1700.14556040757
      | 1671.03347889374
      | 1621.54294032023
      | 1548.76273653566
      | 1513.82823871907
      | 1438.13682678311
      | 1391.55749636099
      | 1339.15574963610
      | 1280.93158660844
      | 1225.61863173217
      | 1176.12809315866
      | 1129.54876273654
      | 1085.880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
  Tq_em [Nm] : Outport
  Q_gen [J/s] : Outport  Port=2
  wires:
  w [rad/s]/1 -> [w], F0009_torque.m/3
  V [V]/1 -> "[0, V_nom]"/1, F0009_torque.m/1, [V]
  I [A]/1 -> F0009_torque.m/2, [I]
  Divide/1 -> "[0,476]"/1
  "[0,476]"/1 -> speed-Torque map1/1
  Constant1/1 -> Divide/2
  [w] -> Divide/1
  "[0, V_nom]"/1 -> Divide/3
  F0009_torque.m/1 -> Torque Limiter/2
  speed-Torque map1/1 -> Gain/1, Torque Limiter/1
  Torque Limiter/1 -> Product/1, Tq_em [Nm]/1
  Gain/1 -> Torque Limiter/3
  [w] -> Product/2
  [V] -> Product1/1
  [I] -> Product1/2
  Product/1 -> Abs1/1
  Product1/1 -> Abs2/1
  Sum/1 -> Abs/1
  Abs/1 -> Q_gen [J/s]/1
  Abs1/1 -> Sum/1
  Abs2/1 -> Sum/2

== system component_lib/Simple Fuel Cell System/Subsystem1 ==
  note: Rolling Fuel Consumption Calculation [kg/100km]
  In1 : Inport
  Add1 : Sum
  Constant6 : Constant
  Constant7 : Constant  Value=100e3
  Demux : Demux
  Divide : Product  Inputs=**/
  Gain1 : Gain  Gain=-1
  Integrator : Integrator
  SC0002_signalRead11 : $bdroot/Data & Control/SC0002_signalRead  SigName=fuelConsumption
  SC0002_signalRead5 : $bdroot/Data & Control/SC0002_signalRead  SigName=hydrogenFlow
  SC0003_signalWrite1 : $bdroot/Data & Control/SC0003_signalWrite  SigName=distance
  Terminator : Terminator
  Terminator1 : Terminator
  Terminator2 : Terminator
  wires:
  Integrator/1 -> Divide/1
  Constant7/1 -> Divide/2
  SC0003_signalWrite1/1 -> Add1/1
  Demux/1 -> Gain1/1
  Add1/1 -> Divide/3
  Constant6/1 -> Add1/2
  Divide/1 -> SC0002_signalRead11/1
  Gain1/1 -> SC0002_signalRead5/1, Integrator/1
  In1/1 -> Demux/1
  Demux/3 -> Terminator1/1
  Demux/4 -> Terminator2/1
  Demux/2 -> Terminator/1

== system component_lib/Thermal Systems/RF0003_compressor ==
  "RF: (h1, p1, ~)" : Inport
  p2 [Pa] : Inport  Port=2
  N [rps] : Inport  Port=3
  Demux : Demux  Outputs=3
  Density Look-up : Lookup_n-D  BreakpointsForDimension1=R1234yf_ph.p  BreakpointsForDimension2=R1234yf_ph.h  Table=R1234yf_ph.D  InternalRulePriority=Speed  RndMeth=Simplest
  Divide : Product  Inputs=*/
  F0021_cp.m : base_lib/F0021_R1234yf/F0021_cp.m  SystemSampleTime=-1  VariantActivationTime=update diagram  Latency=0  AutoFrameSizeCalculation=off
  F0021_cv.m : base_lib/F0021_R1234yf/F0021_cv.m  SystemSampleTime=-1  VariantActivationTime=update diagram  Latency=0  AutoFrameSizeCalculation=off
  F0022_compressor.m : base_lib/F0022_heatPump/F0022_compressor.m  SystemSampleTime=-1  VariantActivationTime=update diagram  Latency=0  AutoFrameSizeCalculation=off
  Gain1 : Gain  Gain=par.M
  Gain2 : Gain  Gain=1/par.M
  Mux : Mux  Inputs=3
  Negative flow barred : Saturate  UpperLimit=inf  LowerLimit=0
  Negative power barred : Saturate  UpperLimit=inf  LowerLimit=0
  Saturation : Saturate  UpperLimit=par.Tc-1  LowerLimit=0
  Temperature Look-up : Lookup_n-D  BreakpointsForDimension1=R1234yf_ph.p  BreakpointsForDimension2=R1234yf_ph.h  Table=R1234yf_ph.T  InternalRulePriority=Speed  RndMeth=Simplest
  Terminator : Terminator
  RF: (h2,p2,W) : Outport
  P_cmp [J/s] : Outport  Port=2
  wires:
  Gain1/1 -> F0022_compressor.m/3, Density Look-up/2, Temperature Look-up/2
  [p_1] -> Temperature Look-up/1, Density Look-up/1, F0022_compressor.m/1
  N [rps]/1 -> F0022_compressor.m/5
  F0022_compressor.m/1 -> Negative flow barred/1
  F0022_compressor.m/2 -> Negative power barred/1
  Density Look-up/1 -> F0022_compressor.m/2, F0021_cv.m/2, F0021_cp.m/2
  F0021_cp.m/1 -> Divide/1
  F0021_cv.m/1 -> Divide/2
  Divide/1 -> F0022_compressor.m/6
  Temperature Look-up/1 -> Saturation/1
  Negative power barred/1 -> P_cmp [J/s]/1
  F0022_compressor.m/3 -> Gain2/1
  p2 [Pa]/1 -> [p_2], F0022_compressor.m/4
  Saturation/1 -> F0021_cv.m/1, F0021_cp.m/1
  Mux/1 -> RF: (h2,p2,W)/1
  Gain2/1 -> [h_2]
  [h_2] -> Mux/1
  [p_2] -> Mux/2
  [W] -> Mux/3
  "RF: (h1, p1, ~)"/1 -> Demux/1
  Demux/1 -> [h_1]
  Demux/2 -> [p_1]
  Demux/3 -> Terminator/1
  [h_1] -> Gain1/1
  Negative flow barred/1 -> [W]

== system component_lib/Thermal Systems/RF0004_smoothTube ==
  "RF: (h1, p1, W1)" : Inport
  Abs : Abs
  Demux : Demux  Outputs=3
  F0021_dliqsat.m : base_lib/F0021_R1234yf/F0021_dliqsat.m  SystemSampleTime=-1  VariantActivationTime=update diagram  Latency=0  AutoFrameSizeCalculation=off
  F0021_dvapsat.m : base_lib/F0021_R1234yf/F0021_dvapsat.m  SystemSampleTime=-1  VariantActivationTime=update diagram  Latency=0  AutoFrameSizeCalculation=off
  F0022_smoothTubePressureDrop.m : base_lib/F0022_heatPump/F0022_smoothTubePressureDrop.m  SystemSampleTime=-1  VariantActivationTime=update diagram  Latency=0  AutoFrameSizeCalculation=off
  Gain{2,4..5,7} (4 alike) : Gain  Gain=par.M
  Mux : Mux  Inputs=3
  R1234yf_mu.m : base_lib/F0021_R1234yf/R1234yf_mu.m  SystemSampleTime=-1  VariantActivationTime=update diagram  Latency=0  AutoFrameSizeCalculation=off
  R1234yf_mu.m1 : base_lib/F0021_R1234yf/R1234yf_mu.m  SystemSampleTime=-1  VariantActivationTime=update diagram  Latency=0  AutoFrameSizeCalculation=off
  R1234yf_sigma.m : base_lib/F0021_R1234yf/R1234yf_sigma.m  SystemSampleTime=-1  VariantActivationTime=update diagram  Latency=0  AutoFrameSizeCalculation=off
  Saturation : Saturate  UpperLimit=par.Tc-1  LowerLimit=0
  Saturation1 : Saturate  UpperLimit=1  LowerLimit=0
  Sum : Sum  Inputs=|+-
  Temperature Look-up : Lookup_n-D  BreakpointsForDimension1=R1234yf_ph.p  BreakpointsForDimension2=R1234yf_ph.h  Table=R1234yf_ph.T  InternalRulePriority=Speed  RndMeth=Simplest
  Vapor Fraction Look-up : Lookup_n-D  BreakpointsForDimension1=R1234yf_ph.p  BreakpointsForDimension2=R1234yf_ph.h  Table=R1234yf_ph.x  InternalRulePriority=Speed  RndMeth=Simplest
  "RF: (h2, p2, W2)" : Outport
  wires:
  Gain2/1 -> Temperature Look-up/2
  [W1] -> Abs/1
  Gain4/1 -> Vapor Fraction Look-up/2
  Vapor Fraction Look-up/1 -> Saturation1/1
  F0021_dvapsat.m/1 -> R1234yf_mu.m1/2, Gain5/1
  Temperature Look-up/1 -> Saturation/1
  Gain5/1 -> F0022_smoothTubePressureDrop.m/4
  F0021_dliqsat.m/1 -> R1234yf_mu.m/2, Gain7/1
  Gain7/1 -> F0022_smoothTubePressureDrop.m/3
  R1234yf_mu.m/1 -> F0022_smoothTubePressureDrop.m/5
  R1234yf_mu.m1/1 -> F0022_smoothTubePressureDrop.m/6
  R1234yf_sigma.m/1 -> F0022_smoothTubePressureDrop.m/7
  [h1] -> Gain4/1, Gain2/1
  Abs/1 -> F0022_smoothTubePressureDrop.m/1
  Demux/2 -> [p1]
  "RF: (h1, p1, W1)"/1 -> Demux/1
  [p1] -> Sum/1
  Sum/1 -> [p2]
  [p1] -> Temperature Look-up/1, Vapor Fraction Look-up/1
  F0022_smoothTubePressureDrop.m/1 -> Sum/2
  Saturation/1 -> R1234yf_sigma.m/1, R1234yf_mu.m1/1, R1234yf_mu.m/1, F0021_dvapsat.m/1, F0021_dliqsat.m/1
  Saturation1/1 -> F0022_smoothTubePressureDrop.m/2
  Mux/1 -> "RF: (h2, p2, W2)"/1
  Demux/1 -> [h1]
  Demux/3 -> [W1]
  [h1] -> Mux/1
  [W1] -> Mux/3
  [p2] -> Mux/2

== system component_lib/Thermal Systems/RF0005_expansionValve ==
  "RF: (h1, p1, W)" : Inport
  exv [-] : Inport  Port=2
  Demux : Demux  Outputs=3
  Density Look-up : Lookup_n-D  BreakpointsForDimension1=R1234yf_ph.p  BreakpointsForDimension2=R1234yf_ph.h  Table=R1234yf_ph.D  InternalRulePriority=Speed  RndMeth=Simplest
  F0021_Tsat.m : base_lib/F0021_R1234yf/F0021_Tsat.m  SystemSampleTime=-1  VariantActivationTime=update diagram  Latency=0  AutoFrameSizeCalculation=off
  F0022_expansionValve.m : base_lib/F0022_heatPump/F0022_expansionValve.m  SystemSampleTime=-1  VariantActivationTime=update diagram  Latency=0  AutoFrameSizeCalculation=off
  Gain : Gain  Gain=1e3
  Gain1 : Gain  Gain=par.M
  Gain2 : Gain  Gain=par.M
  Gain6 : Gain  Gain=par.M
  Integrator : Integrator  InitialCondition=0.9e6
  Mux : Mux  Inputs=3
  Saturation : Saturate  UpperLimit=1  LowerLimit=0
  Saturation1 : Saturate  UpperLimit=par.Tc-1  LowerLimit=0
  Saturation2 : Saturate  UpperLimit=par.pc  LowerLimit=0
  Saturation3 : Saturate  UpperLimit=inf  LowerLimit=p_min
  Sum : Sum  Inputs=|+-
  Sum1 : Sum  Inputs=|+-
  Temperature Look-up : Lookup_n-D  BreakpointsForDimension1=R1234yf_ph.p  BreakpointsForDimension2=R1234yf_ph.h  Table=R1234yf_ph.T  InternalRulePriority=Speed  RndMeth=Simplest
  "RF: (h2, p2, W)" : Outport
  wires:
  Gain2/1 -> Temperature Look-up/2
  Gain1/1 -> Density Look-up/2
  Density Look-up/1 -> Gain6/1
  [W] -> F0022_expansionValve.m/1
  [h_1] -> Gain1/1, Gain2/1
  exv [-]/1 -> Saturation/1
  F0021_Tsat.m/1 -> F0022_expansionValve.m/5
  Gain6/1 -> F0022_expansionValve.m/4
  Saturation/1 -> F0022_expansionValve.m/6
  Temperature Look-up/1 -> Saturation1/1
  Saturation1/1 -> F0022_expansionValve.m/3
  Saturation2/1 -> F0021_Tsat.m/1
  [p_1] -> Saturation2/1, Density Look-up/1, Temperature Look-up/1, F0022_expansionValve.m/2
  "RF: (h1, p1, W)"/1 -> Demux/1
  Demux/2 -> [p_1]
  Demux/1 -> [h_1]
  Demux/3 -> [W]
  Sum/1 -> Saturation3/1
  [dp] -> Sum/2
  [p_1] -> Sum/1
  [h_1] -> Mux/1
  Mux/1 -> "RF: (h2, p2, W)"/1
  [W] -> Mux/3
  Saturation3/1 -> Mux/2
  Sum1/1 -> Gain/1
  F0022_expansionValve.m/1 -> Sum1/1
  Integrator/1 -> Sum1/2, [dp]
  Gain/1 -> Integrator/1
